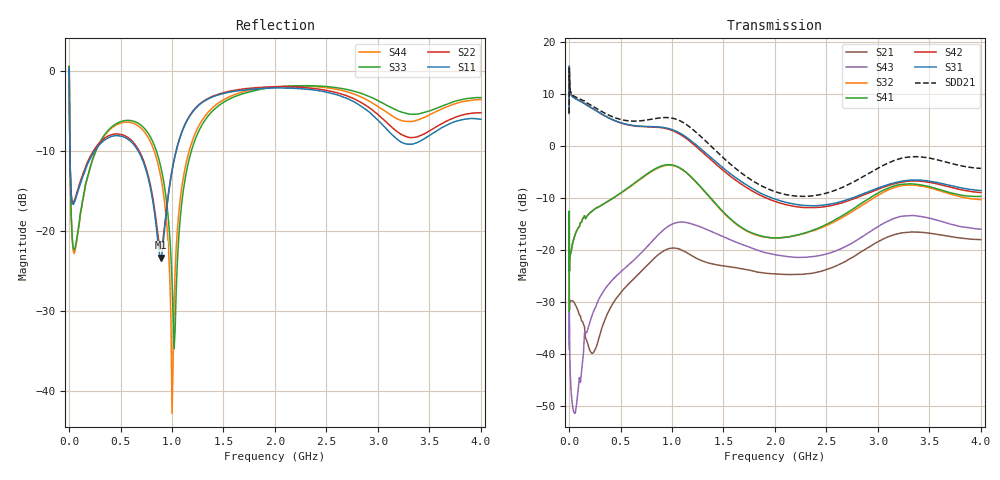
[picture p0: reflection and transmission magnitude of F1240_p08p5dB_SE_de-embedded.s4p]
! Integrated Device Technology
! Corporate Headquarters
! 6024 Silver Creek Valley Road
! San Jose, CA 95138  USA
! Phone:  1-408-284-8200
! Toll Free:  1-800-223-1366
! Webpage:  http://www.idt.com/
! Timing and RF Division
! 515 Groton Road, Suite 102
! Westford, MA 01886-6024
! Device:  F1240
! Description: Dual Intermediate Frequency Digital Variable Gain Amplifier
! Frequency:  10.0 -  500.00 MHz
! Package:  5x5 mm QFN Plastic Package: 32 pin
! Ports:  8 RF, 20 DC
!  Pin  1  = GA3 / Data  Pin 17  = RF OUT_B+
!  Pin  2  = GA4 / CLK  Pin 18  = RF OUT_B-
!  Pin  3  = GA5  Pin 19  = STBY_B
!  Pin  4  = VMODE  Pin 20  = Ground
!  Pin  5  = No Connect  Pin 21  = Ground
!  Pin  6  = GB5  Pin 22  = STB_A
!  Pin  7  = GB4  Pin 23  = RF OUT_A-  = Port 4
!  Pin  8  = GB3  Pin 24  = RF OUT_A+  = Port 3
!  Pin  9  = GB2  Pin 25  = GA0
!  Pin 10  = GB1  Pin 26  = ISET_A
!  Pin 11  = RF IN_B+  Pin 27  = VCC
!  Pin 12  = RF IN_B-  Pin 28  = Ground
!  Pin 13  = Ground  Pin 29  = RF IN_A-  = Port 2
!  Pin 14  = VCC  Pin 30  = RF IN_A+  = Port 1
!  Pin 15  = ISET_B  Pin 31  = GA1
!  Pin 16  = GB0  Pin 32  = GA2 / CSb
! Gain  = +19.5 dB
! State  = 1
! Voltage  = +5.00 V
! Current  = 85.292 mA (one channel only)
! Temperture  =  +25 C
! Test Date  =  2017-10-18
! Board  =  EB4031
! Data:  The device was measured on a custom evaluation board which has
!  individual transmission lines to the RF pins.  Data was collected
!  using a calibrated network analyzer.  The evaluation board was
!  de-embedded using Automatic Fixture Removal.
!  The reference plane is the edge of the package pin.
!  Only Channel A was measured.
!  This data is in single-ended operation.  If your needs are balanced
!  or differential S-parameters then this file needs to be used a
!  linear simulator.
! File Date:  2017-11-10  MJV
! Note:
!  Integrated Device Technology supplies this data as a sample of measured
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# Hz S dB R 100
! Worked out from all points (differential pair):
!   410 points, 500 kHz to 4 GHz, reference 100 ohm
!   strongest paths, dB at 500 kHz, 930 MHz, 1.96 GHz, 2.98 GHz, 4 GHz:
!     S31: 6.2, 3.5, -9.9, -8.2, -8.6
!     S42: 6.2, 3.4, -10.4, -8.5, -9.0
!     S41: -31.8, -3.7, -17.6, -9.3, -9.7
!     S32: -31.3, -3.8, -17.7, -9.7, -10.3
!     S43: -39.0, -15.9, -20.7, -15.8, -16.0
!     S21: -25.6, -20.0, -24.5, -18.6, -18.0
!   taken as a pair (ports 1,2 in; 3,4 out), SDD21 dB: 6.3, 5.4, -8.5, -4.5, -4.3
!   lowest |S11| = -23.4 dB at 890 MHz (marker M1), VSWR 1.15, Z = 112 + j8.53 ohm
!   |S11| at or under -10 dB: 8.41 MHz to 250.4 MHz (242 MHz wide, 187 % of centre); 669.7 MHz to 1.041 GHz (371.6 MHz wide, 43.4 % of centre)
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500000  -0.41 -5.6  -25.54 -4.7  -27.18 82.4  -57.89 71.5
        -25.56 -4.8  -0.40 -5.5  -58.43 70.5  -27.18 83.6
        6.25 -105.1  -31.27 16.4  -0.49 1.4  -39.07 -101.8
        -31.77 13.5  6.22 -103.9  -39.04 -101.4  -0.50 3.7
3000000  -2.58 -61.0  -31.50 -38.9  -15.65 25.9  -56.76 22.3
         -31.50 -37.9  -2.55 -61.0  -57.02 21.3  -15.65 26.1
         14.48 179.0  -20.42 122.4  -2.05 -56.5  -31.03 159.5
         -20.69 120.7  14.48 179.2  -31.03 159.4  -2.11 -56.3
3e7  -16.56 -114.4  -29.66 -12.3  -15.96 -7.8  -45.88 35.9
     -29.71 -12.4  -16.36 -114.5  -45.75 36.7  -15.95 -7.8
     9.51 163.1  -19.12 14.9  -20.74 -101.3  -50.19 105.8
     -19.15 14.5  9.54 163.2  -49.28 110.9  -21.08 -101.2
2e8  -11.14 -140.8  -39.26 -34.6  -17.47 -49.8  -34.40 19.4
     -39.19 -30.7  -10.87 -141.6  -34.37 20.1  -17.49 -49.9
     7.53 110.0  -12.88 -11.0  -12.27 -105.5  -34.60 101.6
     -12.93 -11.6  7.51 109.4  -33.95 98.9  -12.36 -104.4
8.9e8  -23.38 34.2  -20.76 -87.2  -16.51 171.9  -25.75 -140.5
       -20.55 -92.8  -22.29 35.9  -25.95 -133.8  -16.78 171.3
       3.60 -64.6  -4.03 -178.1  -11.96 135.6  -17.43 -70.5
       -3.91 178.2  3.51 -66.3  -16.61 -73.6  -13.22 136.6
1.21e9  -5.00 -113.7  -20.52 -176.2  -18.73 84.0  -25.43 144.3
        -21.27 179.9  -4.94 -113.3  -25.00 151.2  -19.33 82.9
        0.60 -159.2  -6.48 70.2  -9.14 -100.5  -15.61 -168.2
        -6.42 65.4  0.28 -161.0  -15.09 -171.2  -8.33 -104.9
4e9  -6.08 -150.5  -18.11 83.0  -20.36 -66.2  -21.27 -48.1
     -18.00 82.4  -5.26 -147.8  -22.45 -28.5  -22.10 -59.1
     -8.57 21.6  -10.31 -94.7  -3.37 -139.7  -16.92 82.7
     -9.68 -109.0  -8.95 29.3  -15.97 59.2  -3.61 -147.0
